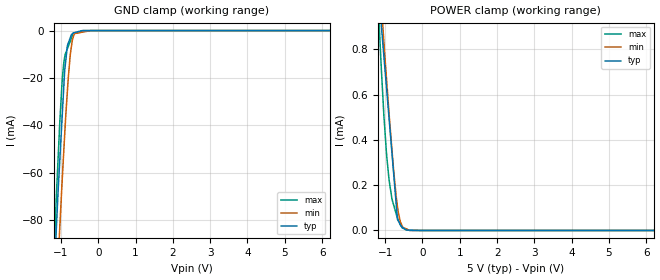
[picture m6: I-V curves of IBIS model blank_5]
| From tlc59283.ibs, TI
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|   blank_5 Model
[Model]   blank_5
Model_type   Input
Vinl = 1.5
Vinh = 3.5
|   typ   min   max
C_comp   5.295e-13   5.058e-13   5.549e-13
| Where nom  PVT is Nominal Process, 5V, 27C
|   Fast PVT is Strong Process,  5.5V, -40C
|   Slow PVT is Weak Process,   4.5V, 125C
[Voltage Range]   5   4.5   5.5
|Ambient Temperature   25   85   -40
|Junction Temperature
[Temperature Range]   27   125   -40
[Power Clamp Reference]   5   4.5   5.5
[GND Clamp Reference]   0   0   0
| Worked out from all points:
|   GND clamp passes 1 mA (typ) near -0.67 V on its own axis
|   POWER clamp passes 1 mA (typ) near -1.15 V on its own axis
[GND Clamp]
|   Voltage   I(typ)   I(min)   I(max)
-5V       -1.681A    -1.606A    -1.772A
-1.238V   -124.2mA   -150.6mA   -112.4mA
-1.14V    -88.92mA   -118.1mA   -75.89mA
-1.122V   -82.82mA   -112.1mA   -69.15mA
-1.034V   -55.24mA   -83.77mA   -39.25mA
-962.5mV  -34.52mA   -61.57mA   -19.98mA
-900mV    -16.8mA    -43.54mA   -11.16mA
-830mV    -6.424mA   -25.93mA   -7.702mA
-751.5mV  -3.024mA   -10.24mA   -4.487mA
-670mV    -966.7uA   -2.507mA   -1.305mA
-202.5mV  -8.64uA    -464.1nA   -3.572uA
10V       0A         0A         0A
[POWER Clamp]
|   Voltage   I(typ)   I(min)   I(max)
-5V       13.71mA    11.48mA    15.23mA
-1.221V   1.234mA    1.281mA    1.114mA
-1.14V    979.4uA    1.086mA    838.7uA
-1.105V   911.1uA    1.003mA    722.3uA
-1.034V   769.5uA    831.2uA    506uA
-968mV    638.8uA    679.5uA    347.5uA
-891mV    486.4uA    506.2uA    218.4uA
-819.5mV  344.8uA    358.9uA    140.6uA
-670mV    48.7uA     104uA      55.32uA
-594mV    26.42uA    38.94uA    24.98uA
-435mV    1.694uA    7.074uA    4.99uA
10V       0A         0A         0A
